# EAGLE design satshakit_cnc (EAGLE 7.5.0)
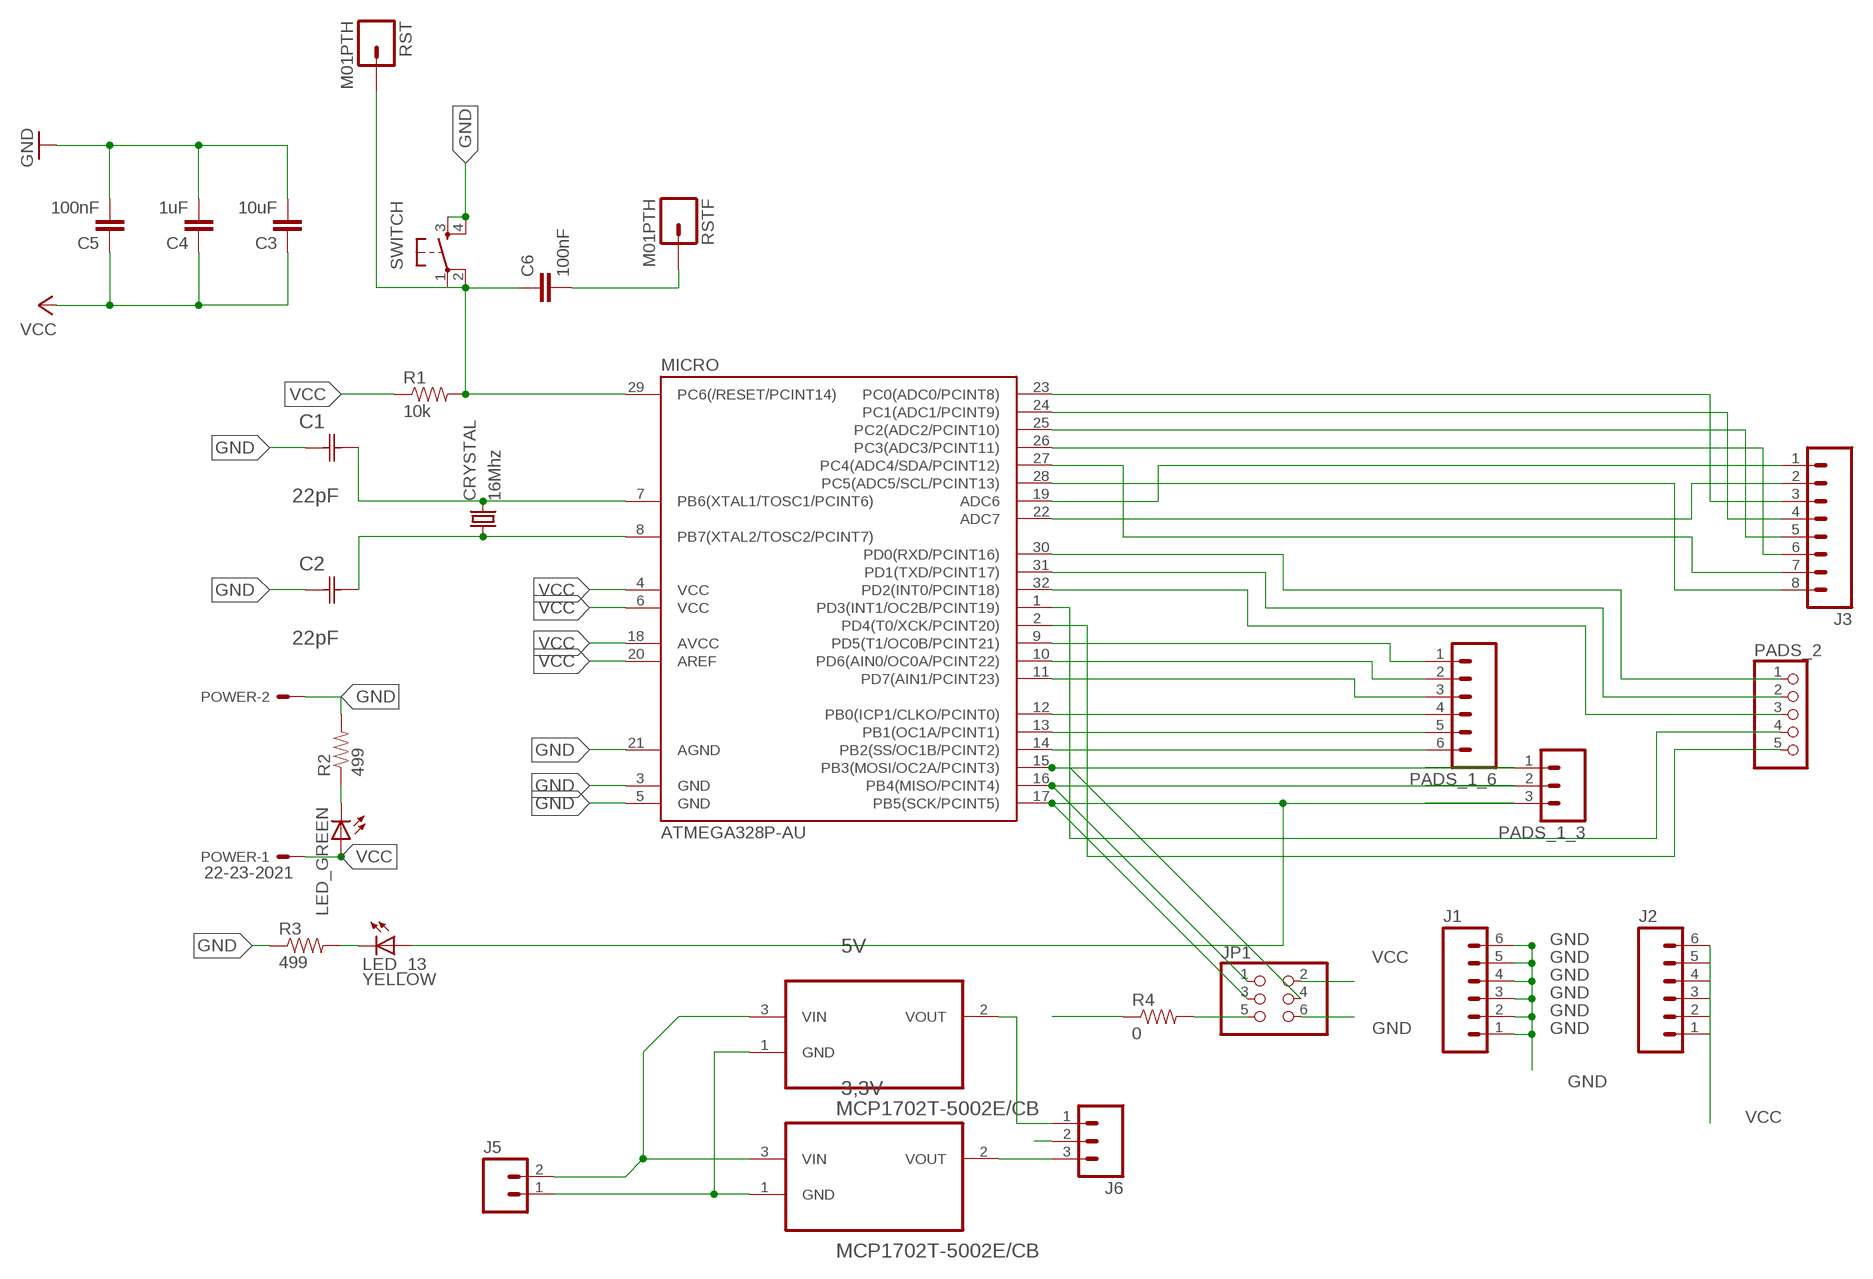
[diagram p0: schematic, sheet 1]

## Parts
3,3V  MCP1702T-5002E/CB  [SOT95P255X145-3N]
5V  MCP1702T-5002E/CB  [SOT95P255X145-3N]
C1  22pF  0612ZC225MAT2A  [CAPC3216X178N]
C2  22pF  0612ZC225MAT2A  [CAPC3216X178N]
C3  10uF  CAP1206  [1206]
C4  1uF  CAP1206  [1206]
C5  100nF  CAP1206  [1206]
C6  100nF  CAP1206  [1206]
CRYSTAL  16Mhz  CSM-7X-DU  [CSM-7X-DU]
J1  M06LONGPADS  [1X06_LONGPADS]
J2  M06LONGPADS  [1X06_LONGPADS]
J3  M08LONGPADS  [1X08_LONGPADS]
J5  M02LOCK_LONGPADS  [1X02_LOCK_LONGPADS]
J6  M03POGO_PIN_HOLES_ONLY  [1X03_PP_HOLES_ONLY]
JP1  PINHD-2X3-SMD  [2X03SMD]
LED_13  YELLOW  LED1206  [1206]
LED_GREEN  LED1206  [1206]
MICRO  ATMEGA328P-AU  ATMEGA48/88/168-AU  [TQFP32-08]
PADS_1_3  M03LONGPADS  [1X03_LONGPADS]
PADS_1_6  M06LONGPADS  [1X06_LONGPADS]
PADS_2  PINHD-1X5  [1X05]
POWER  22-23-2021  [22-23-2021]
R1  10k  RESISTOR1206  [1206]
R2  499  RESISTOR1206  [1206]
R3  499  RESISTOR1206  [1206]
R4  0  RESISTOR1206  [1206]
RST  M01PTH  [1X01]
RSTF  M01PTH  [1X01]
SWITCH  6MM_SWITCH6MM_SWITCH  [6MM_SWITCH]

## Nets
GND: 3,3V.1(GND) 5V.1(GND) C1.1(C1) C2.1(C1) C3.2 C4.2 C5.2 J1.3 J1.4 J1.5 J1.6 J5.1 JP1.6 MICRO.3(GND) MICRO.5(GND) MICRO.21(AGND) POWER.2 R2.2 R3.1 SWITCH.3(S) SWITCH.4(S1)
N$1: MICRO.9(PD5(T1/OC0B/PCINT21)) PADS_1_6.1
N$2: C1.2(C2) CRYSTAL.2 MICRO.7(PB6(XTAL1/TOSC1/PCINT6))
N$3: C6.2 RSTF.1
N$4: MICRO.10(PD6(AIN0/OC0A/PCINT22)) PADS_1_6.2
N$5: MICRO.11(PD7(AIN1/PCINT23)) PADS_1_6.3
N$6: MICRO.12(PB0(ICP1/CLKO/PCINT0)) PADS_1_6.4
N$7: MICRO.13(PB1(OC1A/PCINT1)) PADS_1_6.5
N$8: MICRO.14(PB2(SS/OC1B/PCINT2)) PADS_1_6.6
N$9: C2.2(C2) CRYSTAL.1 MICRO.8(PB7(XTAL2/TOSC2/PCINT7))
N$10: JP1.4 MICRO.15(PB3(MOSI/OC2A/PCINT3)) PADS_1_3.1
N$11: JP1.1 MICRO.16(PB4(MISO/PCINT4)) PADS_1_3.2
N$12: JP1.3 LED_13.1(A) MICRO.17(PB5(SCK/PCINT5)) PADS_1_3.3
N$13: J3.1 MICRO.19(ADC6)
N$14: J3.2 MICRO.22(ADC7)
N$15: J3.3 MICRO.23(PC0(ADC0/PCINT8))
N$16: J3.4 MICRO.24(PC1(ADC1/PCINT9))
N$17: J3.5 MICRO.25(PC2(ADC2/PCINT10))
N$18: J3.6 MICRO.26(PC3(ADC3/PCINT11))
N$19: J3.7 MICRO.27(PC4(ADC4/SDA/PCINT12))
N$20: MICRO.30(PD0(RXD/PCINT16)) PADS_2.1
N$21: MICRO.31(PD1(TXD/PCINT17)) PADS_2.2
N$22: MICRO.32(PD2(INT0/PCINT18)) PADS_2.3
N$23: MICRO.1(PD3(INT1/OC2B/PCINT19)) PADS_2.4
N$24: MICRO.2(PD4(T0/XCK/PCINT20)) PADS_2.5
N$25: J3.8 MICRO.28(PC5(ADC5/SCL/PCINT13))
N$26: LED_GREEN.2(C) R2.1
N$27: LED_13.2(C) R3.2
N$28: JP1.5 R4.2
N$30: 3,3V.3(VIN) 5V.3(VIN) J5.2
N$32: 3,3V.2(VOUT) J6.3
N$33: 5V.2(VOUT) J6.1
RESET: C6.1 MICRO.29(PC6(/RESET/PCINT14)) R1.2 R4.1 RST.1 SWITCH.1(P) SWITCH.2(P1)
VCC: C3.1 C4.1 C5.1 J2.6 J6.2 JP1.2 LED_GREEN.1(A) MICRO.4(VCC) MICRO.6(VCC) MICRO.18(AVCC) MICRO.20(AREF) POWER.1 R1.1
Unconnected: J1.1 J1.2 J2.1 J2.2 J2.3 J2.4 J2.5

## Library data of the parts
3,3V 5V = ldo:MCP1702T-5002E/CB: 250 mA Low Quiescent Current LDO Regulator; MPN: MCP1702T-5002E/CB; OC_FARNELL: 1331491; OC_NEWARK: 84R5180; PACKAGE: SOT23-3; SUPPLIER: Microchip
C1 C2 = AVX_By_element14_Batch_1:0612ZC225MAT2A: Capacitor 1206; MPN: 0612ZC225MAT2A; OC_FARNELL: -; OC_NEWARK: 12N3209; SUPPLIER: AVX; TOLERANCE: ±20%; VALUE: 2.2µF; VOLTAGERATING: 10V
C3-C6 = 01_SparkFun:CAP: Capacitor
CRYSTAL = 01_FAB_Hello:CSM-7X-DU: SMD CRYSTAL; OC_FARNELL: unknown; OC_NEWARK: unknown
J1 J2 PADS_1_6 = SparkFun-Connectors:M06: Header 6 Standard 6-pin 0.1" header. Use with straight break away headers (SKU : PRT-00116), right angle break away headers (PRT-00553), swiss pins (PRT-00743), machine pins (PRT-00117), and female headers (PRT-00115). Molex polarized connector foot print use with SKU : PRT-08094 with associated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
J3 = SparkFun-Connectors:M08: Header 8 Standard 8-pin 0.1" header. Use with straight break away headers (SKU : PRT-00116), right angle break away headers (PRT-00553), swiss pins (PRT-00743), machine pins (PRT-00117), and female headers (PRT-00115).
J5 = SparkFun-Connectors:M02: Standard 2-pin 0.1" header. Use with
J6 PADS_1_3 = SparkFun-Connectors:M03: Header 3 Standard 3-pin 0.1" header. Use with straight break away headers (SKU : PRT-00116), right angle break away headers (PRT-00553), swiss pins (PRT-00743), machine pins (PRT-00117), and female headers (PRT-00115). Molex polarized connector foot print use with SKU : PRT-08232 with associated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
JP1 = fab:PINHD-2X3-SMD: PIN HEADER
LED_13 LED_GREEN = 01_FAB_Hello:LED
MICRO = atmega8:ATMEGA48/88/168
PADS_2 = pinhead:PINHD-1X5: PIN HEADER
POWER = con-molex:22-23-2021: .100" (2.54mm) Center Header - 2 Pin; MF: MOLEX; MPN: 22-23-2021; OC_FARNELL: 1462926; OC_NEWARK: 25C3832
R1-R3 = 01_SparkFun:RESISTOR: Resistor
R4 = SparkFun-Resistors:RESISTOR: Resistor
RST RSTF = 01_SparkFun:M01: Header 1
SWITCH = 01_FAB_Hello:6MM_SWITCH: OMRON SWITCH

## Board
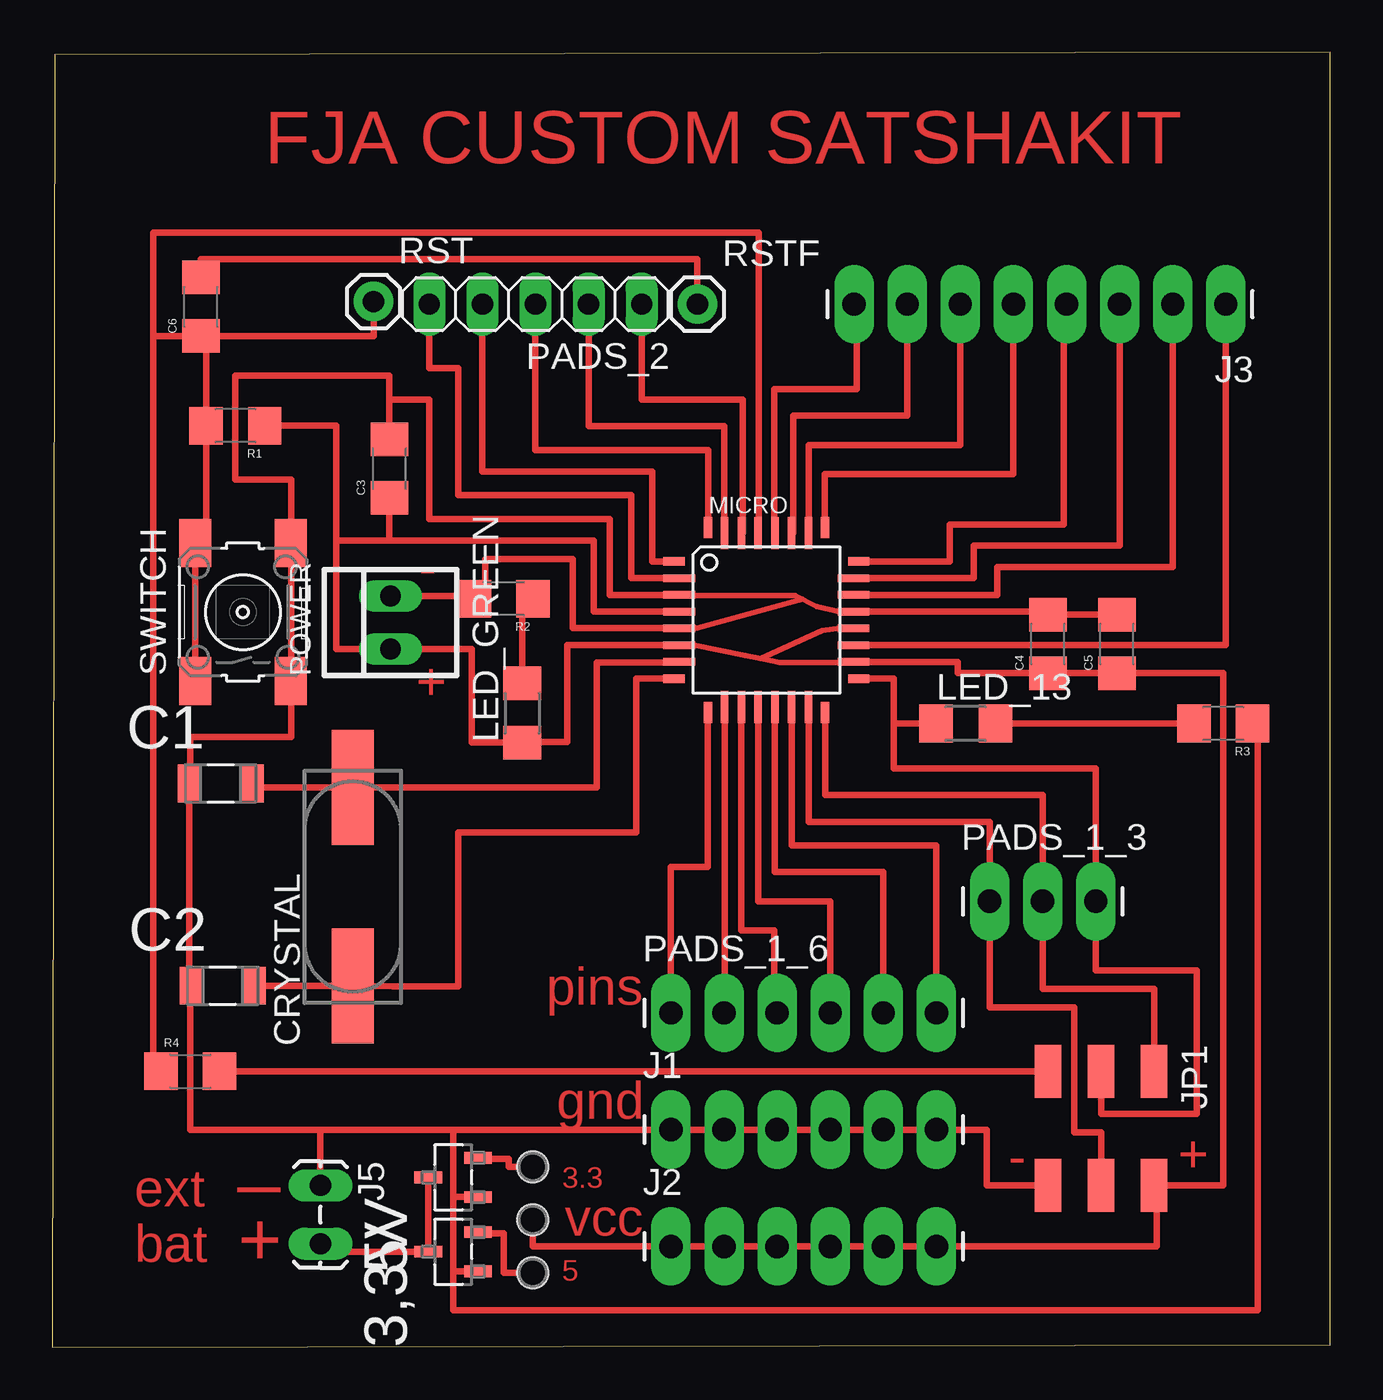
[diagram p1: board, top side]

Size 61.14 x 61.97 mm. Coordinates in mm from the lower left corner, seen from the top.
Outline: 0,0 61.14,0.13 61.14,61.97 0.13,61.84 0,0
Copper layers (1*16): Top 0.035mm / dielectric 1.5mm / Bottom 0.035mm
Design rules "MySettings": minimum track width 6mil, minimum drill 12mil, track to track 6mil, track to pad 6mil, pad to pad 6mil, via to via 6mil, smd to smd 0mil, copper to edge 10mil, drill to drill 10mil, minimum pad ring 10mil, minimum via ring 6mil, stop-mask expansion 2mil, vias tented up to drill 100mil, thermal gap 20mil

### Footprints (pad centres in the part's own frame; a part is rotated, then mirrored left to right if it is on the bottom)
SOT95P255X145-3N = smd 0.559 x 1.321: 1 -0.94,-1.194; 2 0.94,-1.194; 3 0,1.194
CAPC3216X178N = smd 1.118 x 1.803: 1 -1.499,0; 2 1.499,0
1206 = smd 1.6 x 1.8: 1 -1.4,0; 2 1.4,0
CSM-7X-DU = smd 5.5 x 2: 1 -4.75,0; 2 4.75,0
1X06_LONGPADS = drill 1.118 pad 1.88 long: 1 0,0; 2 2.54,0; 3 5.08,0; 4 7.62,0; 5 10.16,0; 6 12.7,0
1X08_LONGPADS = drill 1.118 pad 1.88 long: 1 0,0; 2 2.54,0; 3 5.08,0; 4 7.62,0; 5 10.16,0; 6 12.7,0; 7 15.24,0; 8 17.78,0
1X02_LOCK_LONGPADS = drill 1.016 long: 1 -0.127,0; 2 2.667,0
1X03_PP_HOLES_ONLY = drill 0.9 pad 0.813: 1 0,0; 2 2.54,0; 3 5.08,0 | hole 1.473: 0,0; 2.54,0; 5.08,0
2X03SMD = smd 2.54 x 1.27: 1 -2.54,2.54; 2 2.92,2.54; 3 -2.54,0; 4 2.92,0; 5 -2.54,-2.54; 6 2.92,-2.54
1206' = smd 1.6 x 1.803: 1 -1.422,0; 2 1.422,0
TQFP32-08 = smd 1.016 x 0.406: 1 -4.42,2.8; 8 -4.42,-2.8; 17 4.42,-2.8; 24 4.42,2.8 | smd 1.524 x 0.356: 2 -4.166,2; 3 -4.166,1.2; 4 -4.166,0.4; 5 -4.166,-0.4; 6 -4.166,-1.2; 7 -4.166,-2; 18 4.166,-2; 19 4.166,-1.2; 20 4.166,-0.4; 21 4.166,0.4; 22 4.166,1.2; 23 4.166,2 | smd 0.406 x 1.016: 9 -2.8,-4.42; 16 2.8,-4.42; 25 2.8,4.42; 32 -2.8,4.42 | smd 0.356 x 1.524: 10 -2,-4.166; 11 -1.2,-4.166; 12 -0.4,-4.166; 13 0.4,-4.166; 14 1.2,-4.166; 15 2,-4.166; 26 2,4.166; 27 1.2,4.166; 28 0.4,4.166; 29 -0.4,4.166; 30 -1.2,4.166; 31 -2,4.166
1X03_LONGPADS = drill 1.118 pad 1.88 long: 1 0,0; 2 2.54,0; 3 5.08,0
1X05 = drill 1.016 long: 1 -5.08,0; 2 -2.54,0; 3 0,0; 4 2.54,0; 5 5.08,0
22-23-2021 = drill 1 long: 1 -1.27,0; 2 1.27,0
1X01 = drill 1.016 pad 1.88: 1 0,0
6MM_SWITCH = smd 2.286 x 1.524: 1 -3.302,2.286; 2 3.302,2.286; 3 -3.302,-2.286; 4 3.302,-2.286

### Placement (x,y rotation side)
3,3V  19.18,4.57 90 top
5V  19.18,8.13 90 top
C1  8.05,26.97 0 top
C2  8.15,17.3 0 top
C3  16.13,42.04 90 top
C4  47.62,33.66 90 top
C5  50.93,33.66 90 top
C6  7.11,49.78 90 top
CRYSTAL  14.38,22.05 90 top
J1  29.59,10.41 0 top
J2  29.59,4.83 0 top
J3  56.13,49.91 180 top
J5  12.83,7.62 270 top
J6  22.99,8.64 270 top
JP1  50.16,10.67 270 top
LED_13  YELLOW  [1206']  43.69,29.85 0 top
LED_GREEN  [1206']  22.48,30.35 90 top
MICRO  34.16,34.8 0 top
PADS_1_3  44.83,21.34 0 top
PADS_1_6  29.59,16 0 top
PADS_2  23.11,49.91 180 top
POWER  16.18,34.67 90 top
R1  8.76,44.09 180 top
R2  21.59,35.81 180 top
R3  56.01,29.85 180 top
R4  6.6,13.21 0 top
RST  15.37,50.04 0 top
RSTF  30.86,49.91 0 top
SWITCH  9.12,35.18 90 top

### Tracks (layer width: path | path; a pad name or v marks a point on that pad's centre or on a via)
GND
  Top 0.254: MICRO.3 30.02,35.97 35.55,35.97 | 35.55,35.97 36.58,35.43 37.72,35.18 | 30.61,34.42 30.86,34.42 35.74,35.76 | 35.74,35.76 35.87,35.8 | 35.55,35.97 35.74,35.76
  Top 0.305: MICRO.5 | MICRO.21 | C1.1 6.55,17.3 C2.1 6.6,17.3 6.6,10.41 12.83,10.41 | C1.1 6.48,26.98 | MICRO.5 30,34.42 24.89,34.42 24.89,37.72 20.7,37.72 20.7,35.69 R2.2 20.7,35.94 POWER.2 | C1.1 6.6,26.98 6.6,29.21 11.43,29.21 11.43,31.88 | MICRO.21 47.62,35.2 C4.2 C5.2 | 30.61,34.42 MICRO.5 | MICRO.21 37.72,35.18 | MICRO.3 26.67,36 26.67,39.62 18.03,39.62 18.03,45.34 16.13,45.34 | C3.2 16.13,45.34 | SWITCH.3 11.43,31.88 | 11.43,31.88 11.43,37.85 11.4,37.85 SWITCH.4 11.43,38.48 11.43,41.53 8.76,41.53 8.76,46.48 16.13,46.48 16.13,45.34 | JP1.6 44.7,7.75 44.7,10.41 J1.6 J1.5 J1.4 J1.3 19.18,10.41 | R3.1 57.66,29.85 57.66,1.78 19.18,1.78 19.18,3.63 | 12.83,10.41 19.18,10.41 | 19.18,10.41 19.18,7.19 | 19.18,7.19 19.18,3.68 19.18,3.63 | J5.1 12.83,10.41 | 5V.1 19.18,7.19 | 3,3V.1 19.18,3.63
N$1
  Top 0.305: MICRO.9 31.36,22.99 29.59,22.99 PADS_1_6.1
N$2
  Top 0.305: 9.55,26.8 C1.2 9.55,26.8 | MICRO.7 30,32.77 26.04,32.77 26.04,26.8 CRYSTAL.2 9.55,26.8
N$3
  Top 0.305: RSTF.1 30.86,52.07 7.11,52.07 C6.2
N$4
  Top 0.305: MICRO.10 32.16,20.57 32.16,19.43 32.16,16 PADS_1_6.2
N$5
  Top 0.305: MICRO.11 32.96,19.94 34.54,19.94 34.54,19.81 34.54,16.51 | 34.54,16.51 34.67,16.51 | PADS_1_6.3 34.54,16 34.54,16.51
N$6
  Top 0.305: 33.78,30.63 MICRO.12 33.76,21.34 37.21,21.34 PADS_1_6.4
N$7
  Top 0.305: MICRO.13 34.56,22.73 39.75,22.73 PADS_1_6.5
N$8
  Top 0.305: MICRO.14 35.36,24 42.29,24 PADS_1_6.6
N$9
  Top 0.305: 9.65,17.27 C2.2 | MICRO.8 27.94,32 27.94,24.64 19.43,24.64 19.43,17.27 16.28,17.27 CRYSTAL.1 C2.2 | C2.2
N$10
  Top 0.305: JP1.4 50.16,10.29 48.9,10.29 48.9,16.26 44.83,16.26 PADS_1_3.1 44.83,25.15 36.2,25.15 36.2,30.63 MICRO.15
N$11
  Top 0.305: MICRO.16 36.96,26.42 47.37,26.42 PADS_1_3.2 47.37,17.14 52.7,17.14 JP1.1
N$12
  Top 0.305: 40.26,29.85 40.26,27.69 49.91,27.69 PADS_1_3.3 49.91,18.03 54.74,18.03 54.74,11.18 50.16,11.18 JP1.3 | LED_13.1 40.26,29.85 | MICRO.17 40.26,32 40.26,29.85
N$13
  Top 0.305: MICRO.19 56.13,33.6 J3.1
N$14
  Top 0.305: MICRO.22 45.21,36 45.21,37.34 53.59,37.34 J3.2
N$15
  Top 0.305: MICRO.23 44.07,36.8 44.07,38.35 51.05,38.35 J3.3
N$16
  Top 0.305: MICRO.24 42.93,37.6 42.93,39.37 48.39,39.37 48.39,48.39 48.51,48.39 J3.4
N$17
  Top 0.305: MICRO.25 36.96,41.78 45.97,41.78 J3.5
N$18
  Top 0.305: MICRO.26 36.2,38.96 36.2,43.05 36.2,43.18 43.43,43.18 J3.6
N$19
  Top 0.305: MICRO.27 35.43,38.96 35.43,44.58 40.89,44.58 J3.7
N$20
  Top 0.305: MICRO.30 33.02,38.96 33.02,45.34 28.19,45.34 PADS_2.1
N$21
  Top 0.305: MICRO.31 32.13,38.96 32.13,44.07 25.65,44.07 PADS_2.2
N$22
  Top 0.305: MICRO.32 31.37,42.93 23.11,42.93 PADS_2.3
N$23
  Top 0.305: MICRO.1 28.7,37.6 28.7,41.91 20.57,41.91 PADS_2.4
N$24
  Top 0.305: MICRO.2 27.69,36.8 27.69,40.77 19.43,40.77 19.43,46.86 18.03,46.86 PADS_2.5
N$25
  Top 0.305: MICRO.28 34.54,38.96 34.54,45.72 34.54,45.85 38.48,45.85 38.48,49.91 J3.8
N$26
  Top 0.305: 23.37,35.56 R2.1 22.99,35.43 22.48,35.43 LED_GREEN.2
N$27
  Top 0.305: LED_13.2 R3.2
N$28
  Top 0.305: R4.2 JP1.5
N$30
  Top 0.305: J5.2 12.83,4.57 3,3V.3 5V.3
N$32
  Top 0.305: J6.3 21.59,3.56 21.59,5.46 20.37,5.46 3,3V.2
N$33
  Top 0.305: J6.1 21.84,8.64 21.84,9.02 20.37,9.02 5V.2
RESET
  Top 0.305: R1.2 7.11,44.09 | R1.2 7.36,38.48 SWITCH.2 SWITCH.1 | 7.36,48.38 C6.1 4.83,48.39 | 7.36,48.38 R1.2 | 7.36,48.38 15.37,48.38 RST.1 | MICRO.29 33.78,38.96 33.78,53.34 4.83,53.34 4.83,48.39 | 4.83,48.39 4.83,13.21 R4.1
VCC
  Top 0.254: 30.68,33.6 33.14,33.1 33.9,32.95 | 33.9,32.95 34.8,32.77 38.33,32.77 | MICRO.20 37.72,34.4 37.72,34.42 36.83,34.29 33.9,32.95
  Top 0.305: MICRO.18 | MICRO.20 37.72,34.42 | MICRO.4 25.91,35.2 25.91,38.61 16.13,38.61 | 13.59,38.61 13.59,44.09 R1.1 | 13.59,38.61 13.59,33.4 POWER.1 20.07,33.4 20.07,28.93 LED_GREEN.1 22.48,28.96 24.64,28.96 24.64,33.6 MICRO.6 30.68,33.6 | 38.33,32.77 MICRO.18 | MICRO.18 43.31,32.8 43.31,32.26 C4.1 C5.1 56.01,32.26 56.01,7.75 JP1.2 52.83,7.75 52.83,4.83 J2.6 22.99,4.83 J6.2 | 13.59,38.61 16.13,38.61 | 16.13,38.61 C3.1 16.51,40.64 16.51,40.39

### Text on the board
Top: FJA CUSTOM SATSHAKIT | - | + | pins | gnd | _ | - | + | 3.3 | vcc | ext / bat | + | 5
